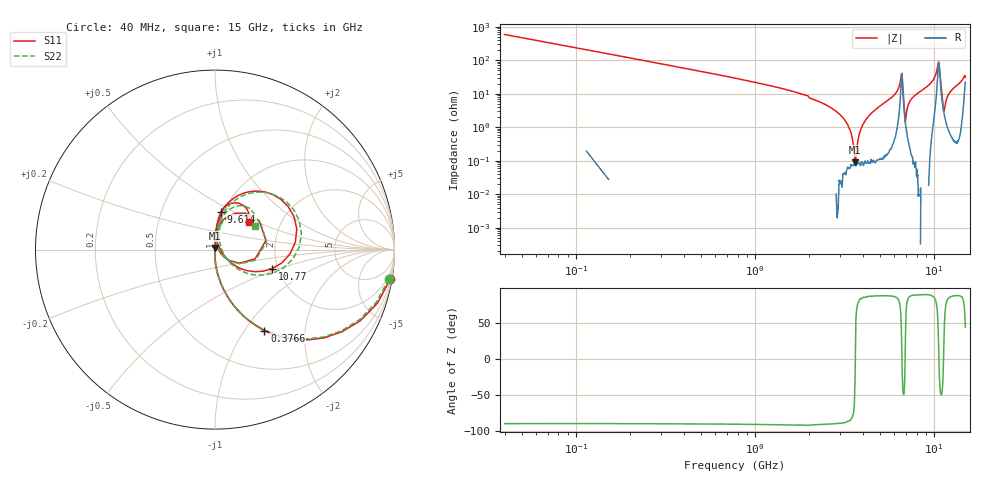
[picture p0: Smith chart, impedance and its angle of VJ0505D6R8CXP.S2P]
! VJ0505D6R8CXP
! MLCC placed on 25 mil thick microstrip substrate in series configuraton.
! DATE 06/29/2018  07:55
! CORRECTED  DATA
# GHz  S  MA  R  50.00
!  FREQ  S11M  S11A  S21M  S21A  S12M  S12A  S22M  S22A
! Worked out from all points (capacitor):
!   401 points, 40 MHz to 15 GHz, reference 50 ohm
!   read as one part in series: C = 6.78 pF near 114.8 MHz
!   lowest |Z| = 90 mohm at 3.63 GHz (marker M1)
!   series resonance near 3.64 GHz, so ESL is about 280 pH
!   S11 on the Smith chart (normalised r, x): 40 MHz: 1, -12; 376.6 MHz: 0.99, -1.24; 9.614 GHz: 0.98, +0.43; 10.77 GHz: 1.86, -0.44; 15 GHz: 1.38, +0.46
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0.04  0.9893 -9.6  0.1684 80.5  0.1686 80.2  0.982 -9.6
0.1896  0.7814 -39.0  0.6293 51.2  0.6297 51.2  0.7746 -39.0
0.3766  0.5289 -58.7  0.8533 31.9  0.8536 31.9  0.5246 -58.4
0.9002  0.2394 -77.1  0.9752 14.0  0.9753 14.1  0.2378 -77.1
2.5458  0.03712 -90.2  0.9989 2.9  0.9996 2.9  0.0368 -88.2
3.0694  0.01268 -93.1  0.9987 1.6  0.9996 1.6  0.01241 -87.8
3.3686  0.001047 -144.6  0.9985 1.0  0.9989 1.0  0.0005923 -10.6
3.6304  0.008481 93.3  0.9984 0.5  0.9989 0.6  0.009001 84.4
4.0792  0.02334 90.1  0.9982 -0.2  0.9986 -0.2  0.02385 87.7
5.0516  0.05619 88.9  0.9964 -1.9  0.9969 -1.9  0.05572 86.1
6.1362  0.1167 83.2  0.9866 -5.2  0.9871 -5.2  0.1161 80.5
6.585  0.2943 33.3  0.7619 -9.9  0.7628 -9.9  0.2959 31.4
6.8842  0.01686 23.1  0.9811 1.2  0.9817 1.2  0.02018 18.8
7.52  0.08364 88.2  0.9942 -3.3  0.9951 -3.3  0.08463 83.9
9.6144  0.2122 80.6  0.9736 -11.0  0.9743 -11.0  0.2179 76.1
10.0258  0.2762 73.7  0.9407 -14.8  0.9421 -14.8  0.2852 69.2
10.4372  0.4271 48.6  0.7598 -22.6  0.7605 -22.6  0.4421 44.7
10.7738  0.3349 -18.4  0.6922 11.7  0.6928 11.8  0.3513 -21.9
11.3348  0.02695 31.2  0.9696 0.4  0.9704 0.4  0.0364 18.2
11.7836  0.07651 85.0  0.9849 -3.4  0.9855 -3.4  0.08025 71.9
12.5316  0.1298 84.7  0.9854 -6.6  0.9861 -6.6  0.1345 78.0
15  0.2453 39.5  0.8054 -10.0  0.8062 -10.0  0.2578 31.3
